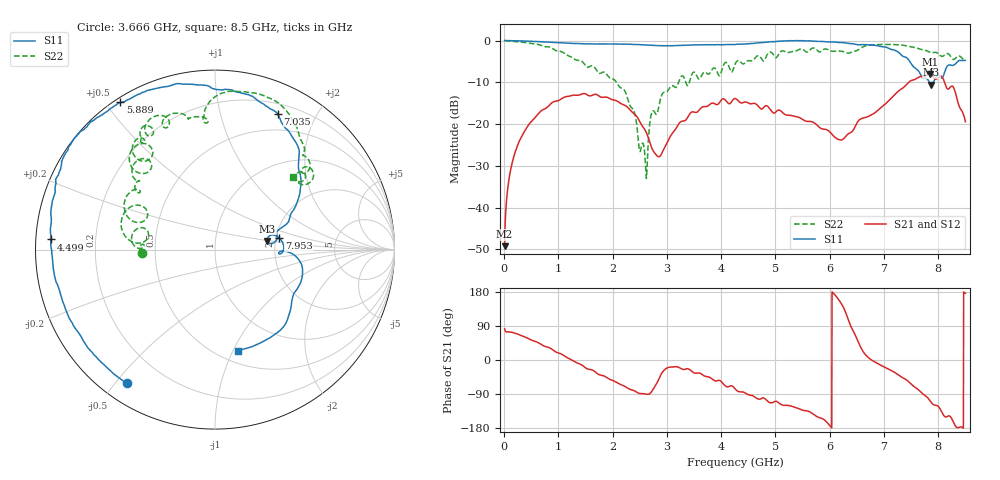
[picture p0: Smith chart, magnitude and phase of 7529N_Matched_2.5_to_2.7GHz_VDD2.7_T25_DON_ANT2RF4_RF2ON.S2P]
!Agilent Technologies,E5071C,MY46417908,A.11.23
!Date: Wed Oct 16 15:59:19 2019
!Data & Calibration Information:
!Freq	S11:SOLT2(ON)	S21:SOLT2(ON)	S12:SOLT2(ON)	S22:SOLT2(ON)
!PortZ  Port1:50+j0  Port2:50+j0
!Above PortZ is port z conversion or system Z0 setting when saving the data.
!When reading, reference impedance value at option line is always used.
# Hz S dB R 50
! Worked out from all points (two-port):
!   1601 points, 10 MHz to 8.5 GHz, reference 50 ohm
!   highest |S21| = -8.07 dB at 7.842 GHz (marker M1); lowest = -49.2 dB at 10 MHz (marker M2)
!   |S21| within 3 dB of the highest: 7.374 GHz to 8.145 GHz (771 MHz wide, 9.94 % of centre); 8.228 GHz to 8.274 GHz (45.97 MHz wide, 0.557 % of centre)
!   lowest |S11| = -10.6 dB at 7.874 GHz (marker M3), VSWR 1.84, Z = 90.6 + j9.54 ohm
!   |S11| at or under -10 dB: 7.838 GHz to 7.911 GHz (73.56 MHz wide, 0.934 % of centre)
!   |S22| runs from -33.0 to -0.1 dB; largest |S21 - S12| = 0.0029
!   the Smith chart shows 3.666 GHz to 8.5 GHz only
!   S11 on the Smith chart (normalised r, x): 3.666 GHz: 0.07, -0.54; 4.499 GHz: 0.04, +0.03; 5.889 GHz: 0.02, +0.55; 7.035 GHz: 0.30, +1.52; 7.953 GHz: 2.09, +0.31; 8.5 GHz: 0.62, -1.05
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1e7  0.01 179.5  -49.25 82.0  -49.34 82.5  -0.06 179.1
1.267375e8  -0.01 173.9  -30.59 73.7  -30.62 73.7  -0.16 172.5
3.602125e8  -0.10 162.6  -22.09 61.9  -22.13 62.0  -0.41 159.7
1.426769e9  -0.74 104.2  -12.84 -12.7  -12.87 -12.6  -4.91 98.4
2.2174e9  -0.85 42.9  -15.47 -68.9  -15.52 -68.8  -11.90 57.0
2.610062e9  -1.05 -0.2  -21.73 -89.8  -21.75 -89.5  -31.03 117.2
2.716188e9  -1.12 -15.1  -25.55 -84.0  -25.56 -83.7  -17.45 -175.1
2.843538e9  -1.22 -34.0  -27.83 -53.0  -27.82 -52.7  -16.31 -168.9
3.19375e9  -1.18 -81.7  -20.44 -18.0  -20.41 -17.8  -10.76 -171.6
3.666006e9  -1.01 -123.4  -15.86 -40.2  -15.83 -40.1  -7.82 -177.1
4.255e9  -0.94 -166.5  -13.88 -75.8  -13.88 -76.2  -5.71 159.5
4.499088e9  -0.75 176.4  -14.93 -91.5  -14.94 -91.9  -4.81 140.0
5.671769e9  -0.11 133.0  -19.45 -140.4  -19.41 -140.3  -1.87 117.5
5.889325e9  -0.22 122.7  -21.21 -156.7  -21.19 -156.6  -2.10 110.9
6.228925e9  -0.46 102.8  -23.76 145.1  -23.76 145.1  -2.56 95.8
7.035475e9  -1.57 65.3  -15.08 -21.0  -15.16 -21.3  -0.91 74.0
7.088538e9  -1.89 62.9  -14.43 -24.3  -14.52 -24.3  -0.92 72.3
7.842025e9  -10.10 6.2  -8.07 -106.3  -8.06 -106.6  -2.78 47.2
7.873862e9  -10.58 9.3  -8.24 -112.4  -8.24 -112.7  -2.88 47.0
7.953456e9  -8.78 10.1  -9.26 -119.4  -9.26 -119.5  -2.81 44.2
8.20285e9  -5.84 -19.8  -11.44 -147.4  -11.43 -147.3  -3.35 36.3
8.5e9  -4.75 -77.1  -19.43 176.2  -19.41 176.6  -4.55 42.8
